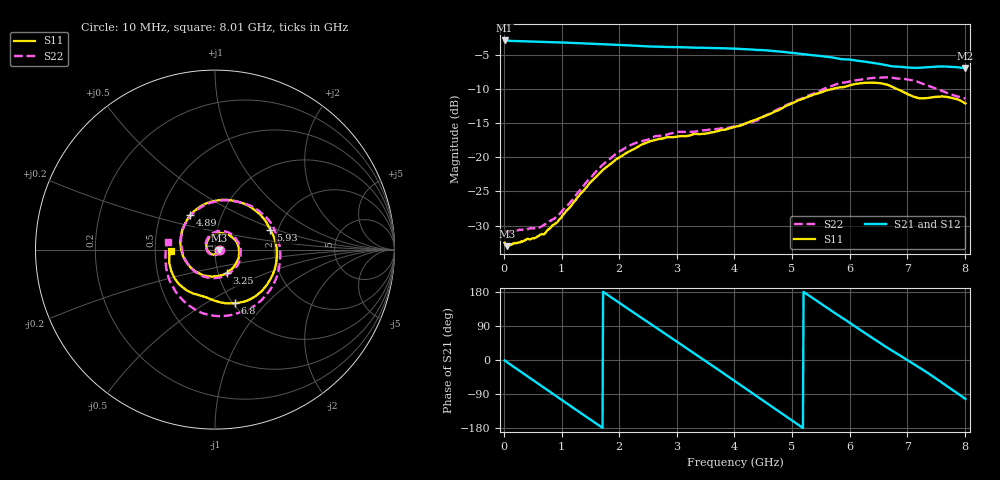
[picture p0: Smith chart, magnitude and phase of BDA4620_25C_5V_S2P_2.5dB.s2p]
!Agilent Technologies,E5071B,MY42404982,A.09.10
!Date: Wed May 06 08:58:36 2026
!Data & Calibration Information:
!Freq	S11:SOLT2(ON)	S21:SOLT2(ON)	S12:SOLT2(ON)	S22:SOLT2(ON)
# Hz S RI R 50
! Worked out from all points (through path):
!   801 points, 10 MHz to 8.01 GHz, reference 50 ohm
!   highest |S21| = -2.94 dB at 10 MHz (marker M1); lowest = -7.0 dB at 8.01 GHz (marker M2)
!   group delay of S21, straight-line fit = 285 ps
!   lowest |S11| = -33.0 dB at 60 MHz (marker M3), VSWR 1.05, Z = 52.3 - j0.32 ohm
!   |S11| at or under -10 dB: start of sweep to 5.718 GHz; 6.814 GHz to end of sweep
!   |S22| runs from -31.0 to -8.3 dB; largest |S21 - S12| = 0.0029
!   S11 on the Smith chart (normalised r, x): 10 MHz: 1.05, -0.00; 3.25 GHz: 1.10, -0.29; 4.89 GHz: 0.71, +0.29; 5.93 GHz: 1.82, +0.45; 6.8 GHz: 1.02, -0.68; 8.01 GHz: 0.60, -0.01
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1e7  0.0236 -0.00168  0.7127 -0.0152  0.7136 -0.0154  0.0294 -0.00196
6e7  0.0222 -0.00306  0.7049 -0.0816  0.7065 -0.0827  0.0279 -0.00358
3.6e8  0.0178 -0.017  0.5521 -0.4348  0.5524 -0.4359  0.0215 -0.0201
7.3e8  -0.00676 -0.0277  0.1559 -0.6775  0.1556 -0.6785  -0.00656 -0.032
1.03e9  -0.0356 -0.0137  -0.2168 -0.6525  -0.2175 -0.6534  -0.0381 -0.0163
1.35e9  -0.0481 0.0271  -0.5338 -0.4208  -0.5341 -0.4212  -0.0527 0.0277
1.64e9  -0.0273 0.0698  -0.6643 -0.0957  -0.6652 -0.0959  -0.0327 0.075
1.93e9  0.0219 0.0926  -0.6154 0.2455  -0.6164 0.2461  0.0199 0.1028
2.32e9  0.0979 0.0669  -0.3053 0.5751  -0.3065 0.5756  0.1032 0.0765
2.68e9  0.1354 -0.00937  0.0966 0.6345  0.0971 0.6351  0.143 0.00209
3.25e9  0.0669 -0.1292  0.5823 0.2452  0.5836 0.2446  0.0845 -0.1281
3.62e9  -0.0265 -0.1497  0.6054 -0.1653  0.6057 -0.1667  -0.0168 -0.1595
4.01e9  -0.1293 -0.1049  0.3472 -0.5141  0.347 -0.5152  -0.1295 -0.1077
4.44e9  -0.1916 0.0233  -0.1141 -0.5958  -0.1158 -0.5966  -0.1872 0.0313
4.89e9  -0.139 0.1908  -0.4982 -0.3085  -0.4984 -0.3088  -0.1134 0.21
5.35e9  0.0605 0.2775  -0.5357 0.1502  -0.5358 0.1505  0.0999 0.2706
5.93e9  0.3087 0.1095  -0.1391 0.4997  -0.1388 0.5011  0.3432 0.0777
6.27e9  0.3377 -0.09  0.1638 0.4708  0.1649 0.4709  0.3533 -0.1205
6.68e9  0.1765 -0.2854  0.4037 0.2329  0.4053 0.2329  0.2056 -0.3233
6.8e9  0.1098 -0.2984  0.4347 0.1491  0.4363 0.1488  0.1356 -0.3513
7.36e9  -0.1037 -0.2503  0.3744 -0.2577  0.375 -0.259  -0.1807 -0.2803
8.01e9  -0.2469 -0.00529  -0.0968 -0.4371  -0.0974 -0.4381  -0.2644 0.045
